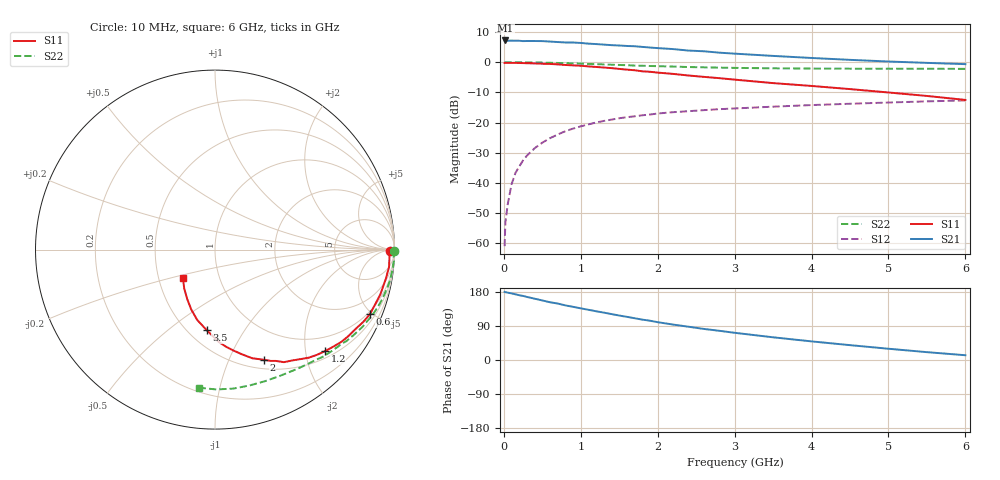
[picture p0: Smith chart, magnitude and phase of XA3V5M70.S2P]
! SIEMENS Discrete & RF Semiconductors
! BFY180
! Si NPN RF Bipolar Junction Transistor in MICRO-X
! VCE = 3.5 V  IC = 0.7 mA
! Common Emitter S-Parameters:  May  1997
# GHz  S  MA  R  50
!  f  S11  S21  S12  S22
! GHz  MAG  ANG  MAG  ANG  MAG  ANG  MAG  ANG
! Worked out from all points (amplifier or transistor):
!   36 points, 10 MHz to 6 GHz, reference 50 ohm
!   highest |S21| = 7.2 dB at 20 MHz (marker M1)
!   |S21| within 3 dB of that: start of sweep to 2.259 GHz
!   unconditionally stable (mu >= 1): 4.644 GHz to end of sweep
!   at 250 MHz: K = 0.07, MSG = 19.7 dB, |S12| = -32.5 dB
!   at 1.4 GHz: K = 0.43, MSG = 12.3 dB, |S12| = -19.0 dB
!   at 6 GHz: K = 1.04, MAG = 4.8 dB, |S12| = -12.7 dB
!   S11 on the Smith chart (normalised r, x): 10 MHz: 69, -13; 600 MHz: 0.85, -4.86; 1.2 GHz: 0.65, -2.40; 2 GHz: 0.61, -1.36; 3.5 GHz: 0.61, -0.69; 6 GHz: 0.67, -0.22
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0.01  0.9724 -0.3  2.261 179.7  0.0009 89.7  0.9972 -0.3
0.02  0.9729 -0.7  2.289 179.0  0.0022 85.2  0.9999 -0.5
0.05  0.9725 -1.9  2.265 177.8  0.0044 87.0  0.9979 -1.2
0.1  0.9733 -3.9  2.274 175.7  0.0095 88.2  0.9959 -2.4
0.15  0.9745 -5.8  2.267 173.4  0.0146 86.1  0.9982 -3.7
0.3  0.9611 -11.4  2.242 166.4  0.0284 81.9  0.9928 -7.3
0.5  0.9429 -18.9  2.233 157.2  0.0465 76.3  0.9847 -12.1
0.6  0.9353 -22.6  2.194 152.4  0.0552 73.5  0.9774 -14.4
0.9  0.8855 -33.0  2.117 140.3  0.0795 65.4  0.9549 -21.2
1.1  0.8517 -39.5  2.028 132.5  0.0934 60.4  0.9363 -25.4
1.2  0.8335 -42.8  1.994 128.6  0.1004 58.2  0.9285 -27.5
1.5  0.7742 -52.0  1.89 117.3  0.118 51.9  0.8996 -33.2
1.7  0.7356 -58.5  1.836 110.2  0.127 48.4  0.8781 -36.8
2  0.672 -66.0  1.71 99.8  0.1413 43.4  0.8591 -41.7
2.2  0.6398 -71.1  1.648 93.5  0.1487 40.0  0.8461 -45.0
2.6  0.5713 -79.7  1.516 82.0  0.1608 35.1  0.8213 -50.7
3  0.5142 -87.8  1.385 71.8  0.1713 30.4  0.8047 -56.2
3.5  0.4505 -96.0  1.27 59.9  0.1835 25.7  0.7914 -62.6
4  0.4042 -104.2  1.174 49.1  0.195 21.0  0.7844 -69.1
4.5  0.3585 -111.7  1.093 39.2  0.205 16.9  0.7811 -75.7
5.5  0.2761 -128.4  0.974 20.7  0.2245 8.5  0.7791 -89.5
6  0.2373 -139.0  0.928 12.6  0.2327 4.2  0.7748 -96.4
